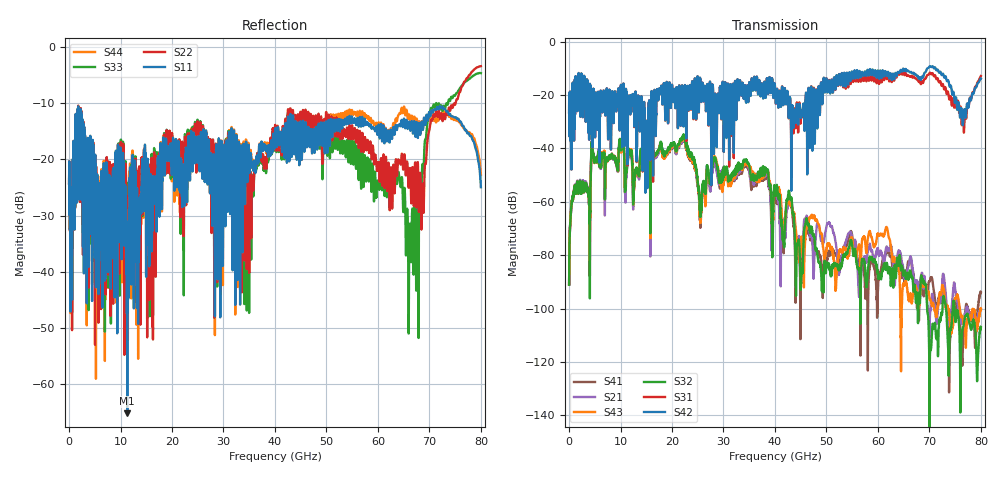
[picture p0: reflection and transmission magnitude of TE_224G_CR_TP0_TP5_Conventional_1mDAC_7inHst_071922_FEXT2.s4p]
!! Reference: tracy_3df_01a_2207
!! CHANNEL DESCRIPTION: TP0_TP5 CR Channel using 1meter DAC, Conventional 7in Host
!! MODEL DESCRIPTION: s4p, FEXT2
!! CONNECTOR DESCRIPTION: OSFP 200G SMT
!! CABLE DESCRIPTION: 1meter 26AWG Cable
!! MODEL STATUS: Developmental
!! PORT DEFINITIONS:
!! Port  1  ----->  Side A  Side B  <-----  Port  2
!! Port  3  ----->  Side A  Side B  <-----  Port  4
# GHz S MA R 50
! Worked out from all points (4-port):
!   8000 points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, 10 MHz to 80 GHz, reference 50 ohm
!   strongest paths, dB at 10 MHz, 20.01 GHz, 40.01 GHz, 60.01 GHz, 80 GHz:
!     S42: -26.6, -16.2, -17.4, -11.0, -13.9
!     S31: -26.6, -16.2, -17.4, -12.4, -12.9
!     S32: -91.1, -38.8, -55.9, -87.3, -107.0
!     S43: -91.0, -39.3, -57.4, -72.0, -100.2
!     S21: -90.8, -39.7, -57.4, -77.8, -100.4
!     S41: -91.1, -40.0, -59.3, -92.8, -94.0
!   lowest |S11| = -65.2 dB at 11.3 GHz (marker M1), VSWR 1.00, Z = 50 - j0.0496 ohm
!   |S11| at or under -10 dB: start of sweep to end of sweep
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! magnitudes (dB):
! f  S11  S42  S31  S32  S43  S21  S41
! 10 MHz  -24.3  -26.6  -26.6  -91.1  -91.0  -90.8  -91.1
! 4.65 GHz  -25.0  -25.8  -25.8  -42.0  -42.3  -41.9  -42.2
! 11.3 GHz  -65.2  -29.0  -29.0  -46.1  -45.7  -47.1  -46.4
! 22.26 GHz  -23.2  -26.2  -26.0  -34.8  -35.1  -35.9  -36.1
! 46.19 GHz  -17.9  -25.7  -24.3  -66.5  -68.8  -65.4  -67.9
! 66.19 GHz  -14.0  -11.5  -13.1  -85.7  -95.2  -81.3  -81.6
! 80 GHz  -24.9  -13.9  -12.9  -107.0  -100.2  -100.4  -94.0
